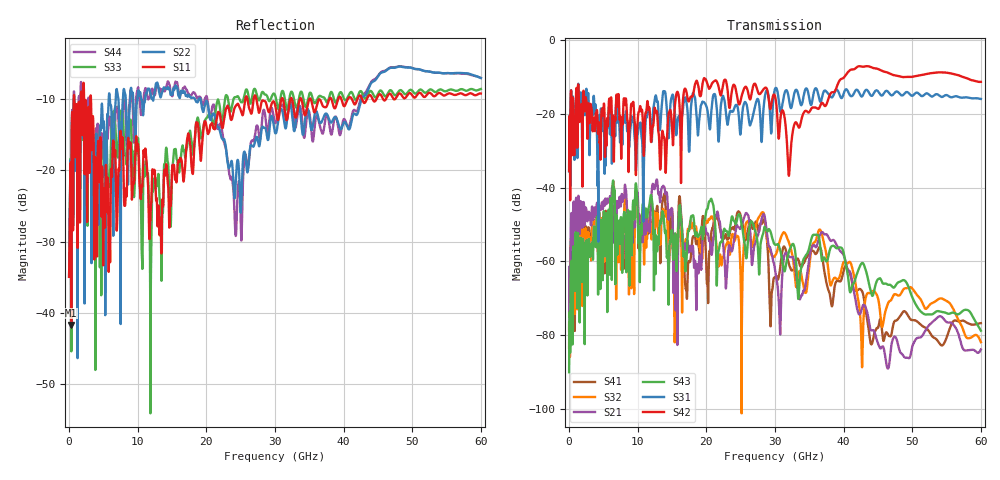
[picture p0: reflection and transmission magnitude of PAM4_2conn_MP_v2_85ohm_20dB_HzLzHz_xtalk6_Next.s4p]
! Info: Touchstone file created by Circ.  Input file=FAB50GbE_2conn_Midplane_Examax_Topo2_v2_85ohm_20dB_HzLzHz.circ
# Hz S RI R 50
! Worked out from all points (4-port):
!   6000 points, 10 MHz to 60 GHz, reference 50 ohm
!   strongest paths, dB at 10 MHz, 15.01 GHz, 30.01 GHz, 45.01 GHz, 60 GHz:
!     S42: -35.5, -24.0, -15.3, -7.9, -11.4
!     S31: -35.6, -15.1, -13.3, -13.9, -16.0
!     S43: -90.0, -51.7, -55.5, -64.8, -78.8
!     S21: -78.2, -46.0, -62.3, -82.2, -83.9
!     S32: -78.9, -52.3, -58.4, -70.0, -81.9
!     S41: -83.5, -46.0, -64.3, -78.0, -76.7
!   lowest |S11| = -41.7 dB at 320 MHz (marker M1), VSWR 1.02, Z = 49.4 + j0.526 ohm
!   |S11| at or under -10 dB: 3.193 GHz to 25.68 GHz (22.49 GHz wide, 156 % of centre); 27.28 GHz to 30.94 GHz (3.658 GHz wide, 12.6 % of centre); 35.2 GHz to 37.92 GHz (2.713 GHz wide, 7.42 % of centre)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
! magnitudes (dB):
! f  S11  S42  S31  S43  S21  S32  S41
! 10 MHz  -34.9  -35.5  -35.6  -90.0  -78.2  -78.9  -83.5
! 320 MHz  -41.7  -14.1  -13.9  -60.5  -47.7  -54.8  -53.8
! 12.59 GHz  -22.1  -19.4  -15.2  -60.5  -39.3  -50.0  -47.0
! 20.64 GHz  -13.6  -12.7  -21.6  -43.2  -56.5  -48.0  -55.0
! 32.06 GHz  -10.9  -36.5  -16.3  -57.2  -58.8  -55.1  -60.9
! 42.09 GHz  -9.8  -7.2  -13.8  -62.7  -73.7  -70.0  -67.7
! 60 GHz  -9.2  -11.4  -16.0  -78.8  -83.9  -81.9  -76.7
